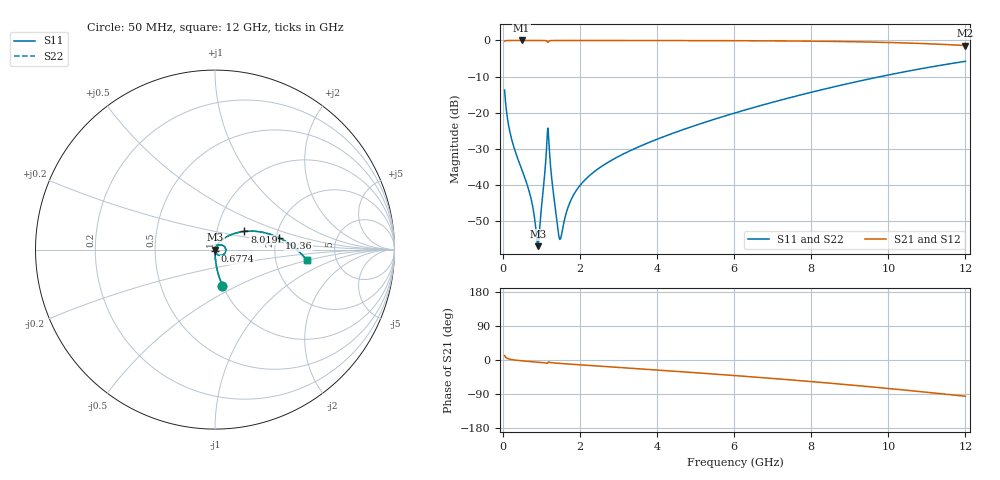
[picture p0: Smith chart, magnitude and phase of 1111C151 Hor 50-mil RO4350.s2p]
# GHz S MA R 50
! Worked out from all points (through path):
!   1601 points, 50 MHz to 12 GHz, reference 50 ohm
!   highest |S21| = -0.01 dB at 490.7 MHz (marker M1); lowest = -1.4 dB at 12 GHz (marker M2)
!   group delay of S21, straight-line fit = 22 ps
!   lowest |S11| = -56.9 dB at 908.9 MHz (marker M3), VSWR 1.00, Z = 50.1 - j0.0394 ohm
!   |S11| at or under -10 dB: start of sweep to 9.796 GHz
!   |S22| runs from -56.9 to -5.8 dB; largest |S21 - S12| = 0
!   S11 on the Smith chart (normalised r, x): 50 MHz: 1.00, -0.42; 677.4 MHz: 1.00, -0.02; 8.019 GHz: 1.36, +0.29; 10.36 GHz: 2.08, +0.31; 12 GHz: 3.03, -0.48
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0.05  0.2061 -78.3  0.9782 11.6  0.9782 11.6  0.2061 -78.3
0.2143125  0.04715 -87.9  0.9983 1.4  0.9983 1.4  0.04715 -87.9
0.4906563  0.01669 -89.0  0.999 -2.0  0.999 -2.0  0.01669 -89.0
0.677375  0.008548 -86.6  0.9989 -3.6  0.9989 -3.6  0.008548 -86.6
0.8715625  0.002137 -57.4  0.9986 -5.2  0.9986 -5.2  0.002137 -57.4
0.9089063  0.001432 -15.9  0.9985 -5.5  0.9985 -5.5  0.001432 -15.9
0.9611875  0.002606 45.5  0.9983 -6.0  0.9983 -6.0  0.002606 45.5
1.1255  0.02522 55.8  0.9886 -8.2  0.9886 -8.2  0.02522 55.8
1.170313  0.06136 -1.8  0.9389 -7.5  0.9389 -7.5  0.06136 -1.8
1.215125  0.02816 -66.3  0.9857 -6.0  0.9857 -6.0  0.02816 -66.3
1.289813  0.0101 -77.3  0.9964 -7.3  0.9964 -7.3  0.0101 -77.3
1.409312  0.003053 -58.2  0.9979 -8.4  0.9979 -8.4  0.003053 -58.2
1.484  0.001776 -7.3  0.9981 -9.0  0.9981 -9.0  0.001776 -7.3
1.745406  0.005804 62.6  0.9982 -10.9  0.9982 -10.9  0.005804 62.6
2.044156  0.01048 67.7  0.9981 -13.0  0.9981 -13.0  0.01048 67.7
2.783562  0.02144 66.8  0.9977 -18.0  0.9977 -18.0  0.02144 66.8
4.038312  0.0438 60.2  0.9964 -26.7  0.9964 -26.7  0.0438 60.2
6.025  0.09946 47.1  0.9916 -41.1  0.9916 -41.1  0.09946 47.1
8.019156  0.193 31.7  0.9766 -57.1  0.9766 -57.1  0.193 31.7
10.01331  0.3339 13.8  0.9367 -75.3  0.9367 -75.3  0.3339 13.8
10.36434  0.3635 10.4  0.9255 -78.7  0.9255 -78.7  0.3635 10.4
12  0.5143 -6.4  0.8503 -95.7  0.8503 -95.7  0.5143 -6.4
